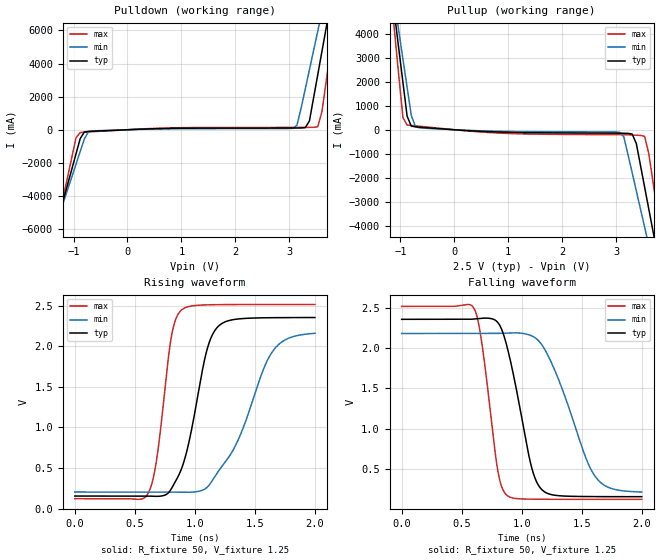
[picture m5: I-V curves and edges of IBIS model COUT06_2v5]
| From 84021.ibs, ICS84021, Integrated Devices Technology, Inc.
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[Model] COUT06_2v5
Model_type   Output
Polarity   Non-Inverting
|   typ   min   max
C_comp   2pF   1.5pF   2.5pF
Vmeas = 1.25V
Rref = 50
Vref = 1.25V
|   typ   min   max
[Voltage range]   2.5V   2.375V   2.625V
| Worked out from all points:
|   slope of the pulldown table from 0 to 0.375 V, typ, clamps not added: 7.84 ohm
|   slope of the pullup table from 0 to 0.375 V, typ, clamps not added: 7.16 ohm
|   rising waveform, R_fixture 50, V_fixture 1.25: 20-80 % time 181ps typ, 322ps min, 114ps max; typ from 0.154 V to 2.35 V
|   falling waveform, R_fixture 50, V_fixture 1.25: 20-80 % time 175ps typ, 285ps min, 118ps max; typ from 2.35 V to 0.154 V
[pulldown]
|Voltage   I (typ)   I (min)   I (max)
-2.5V     -19.75A    -17.31A    -23.85A
-1.34V    -6.031A    -5.882A    -6.333A
-953.6mV  -1.449A    -2.071A    -479.4mA
-876.3mV  -533mA     -1.309A    -169.7mA
-644.3mV  -89.97mA   -69.78mA   -117.4mA
3.067V    103.7mA    87.56mA    139.5mA
3.144V    104.2mA    267.1mA    139.8mA
3.376V    532mA      3.625A     142.7mA
3.531V    3.329A     5.955A     178.4mA
3.686V    6.13A      8.286A     2.887A
3.84V     8.933A     10.62A     6.471A
5V        29.99A     28.14A     33.4A
[pullup]
|Voltage   I (typ)   I (min)   I (max)
-2.5V     30.11A     26.36A     36.43A
-1.108V   4.788A     5.285A     4.064A
-1.031V   3.38A      4.114A     2.264A
-953.6mV  1.972A     2.943A     504.8mA
-876.3mV  566.5mA    1.772A     199.4mA
-799mV    152.8mA    600.7mA    177mA
3.067V    -143.2mA   -109.6mA   -206.5mA
3.299V    -177.9mA   -1.786A    -218.7mA
3.531V    -2.395A    -4.061A    -274.9mA
3.686V    -4.221A    -5.58A     -2.168A
3.84V     -6.047A    -7.1A      -4.502A
5V        -19.75A    -18.51A    -22.01A
[Ramp]
|   typ   min   max
dV/dt_r   1.50/0.6n   1.50/0.80n   1.50/0.4n
dV/dt_f   1.50/0.6n   1.50/0.80n   1.50/0.4n
[Rising Waveform]
R_fixture = 50
V_fixture = 1.25
V_fixture_max = 1.3125
V_fixture_min = 1.1875
C_fixture = 0.0p
0s        154.1mV    203.2mV    121.3mV
609ps     154.1mV    203.2mV    184mV
682.5ps   150.3mV    203.3mV    612.2mV
806.4ps   249.2mV    203.4mV    2.136V
892.5ps   505.9mV    202.2mV    2.452V
1.094ns   1.919V     251.9mV    2.51V
1.184ns   2.23V      435mV      2.513V
1.359ns   2.337V     840.1mV    2.515V
1.646ns   2.353V     1.935V     2.515V
1.999ns   2.355V     2.16V      2.515V
[Falling Waveform]
R_fixture = 50
V_fixture = 1.25
V_fixture_max = 1.3125
V_fixture_min = 1.1875
C_fixture = 0.0p
0s        2.355V     2.179V     2.515V
602.7ps   2.358V     2.179V     2.489V
665.7ps   2.367V     2.179V     2.08V
802.2ps   2.313V     2.18V      463.4mV
877.8ps   2.013V     2.185V     169.6mV
1.073ns   571.7mV    2.155V     123.2mV
1.161ns   250.7mV    2.051V     122mV
1.296ns   167.9mV    1.648V     121.4mV
1.606ns   155.1mV    416.2mV    121.3mV
1.999ns   154.1mV    211.8mV    121.3mV
